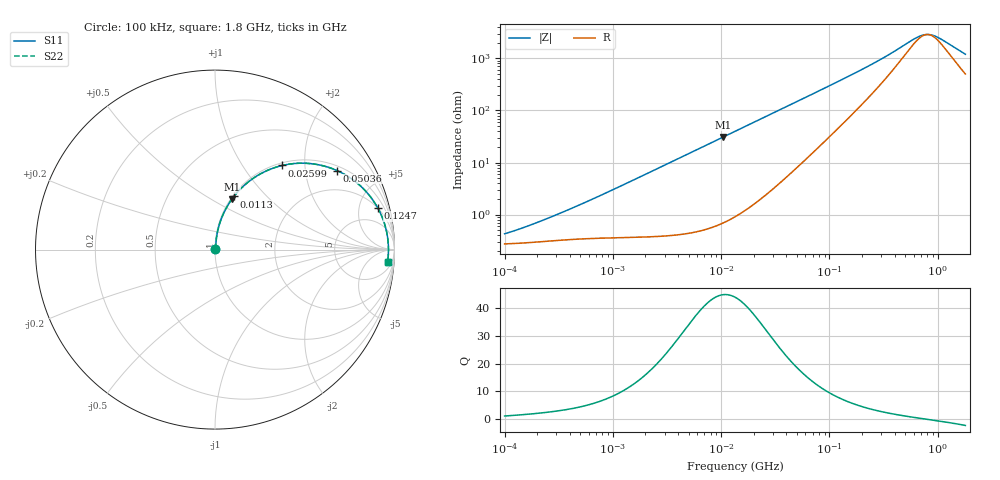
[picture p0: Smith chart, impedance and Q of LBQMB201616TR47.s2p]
! LBQMB201616TR47  S-PARAMETER MODEL  ( General Type )
! Model Generated by TAIYO YUDEN Corporation (http://www.ty-top.com)
! Version 1.0
! TAIYO YUDEN Control No. 191025NI43SB-FBB
! Copyright(c) 2019 TAIYO YUDEN CO.,LTD. All Rights Reserved.
! Product Description (link to TY-COMPAS)
! https://ds.yuden.co.jp/TYCOMPAS/or/detail?pn=LBQMB201616TR47J&u=M
! Products Name : Inductors
! Characteristics :
!  Inductance : 0.47 uH , SRF(min) : 350 MHz , DC Resistance(max) : 0.338 Ohm , Rated Current : 430 mA
!  Case Size : 2.0 x 1.6 / 0.079 x 0.063 [mm/inch] , Thickness : 1.6 / 0.063 [mm/inch]
!  (Conditions: Temperature = 25 degC , DC Bias Current/Voltage = 0A / 0V)
! External Node Assignments :
!  1  o---GGG---o  2
! GND o---------o GND
! Frequency Range : 0.1MHz  -  1800MHz  [ 402 STEP ]
# MHz S RI R 50
! Freq[MHz].  S11 Real  S11 Imag  S21 Real  S21 Imag  S12 Real  S12 Imag  S22 Real  S22 Imag
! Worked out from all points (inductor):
!   401 points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, 100 kHz to 1.8 GHz, reference 50 ohm
!   read as one part in series: L = 489 nH near 308.6 kHz
!   highest Q = 44.7 at 10.5 MHz (marker M1), where L = 470 nH
!   self-resonance near 803.5 MHz
!   S11 on the Smith chart (normalised r, x): 100 kHz: 1.01, +0.01; 11.3 MHz: 1.01, +0.67; 25.99 MHz: 1.05, +1.54; 50.36 MHz: 1.16, +2.98; 124.7 MHz: 1.98, +7.42; 1.8 GHz: 11, -22
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0.1  0.00273 0.00327  0.9973 -0.00327  0.9973 -0.00327  0.00273 0.00327
0.193745  0.00298 0.00616  0.997 -0.00616  0.997 -0.00616  0.00298 0.00616
0.516129  0.00363 0.0155  0.9964 -0.0155  0.9964 -0.0155  0.00363 0.0155
2.66389  0.00989 0.0777  0.9901 -0.0777  0.9901 -0.0777  0.00989 0.0777
5.420303  0.0291 0.1547  0.9709 -0.1547  0.9709 -0.1547  0.0291 0.1547
10.50158  0.0929 0.2794  0.9071 -0.2794  0.9071 -0.2794  0.0929 0.2794
11.30236  0.1056 0.2963  0.8944 -0.2963  0.8944 -0.2963  0.1056 0.2963
13.41641  0.1414 0.3372  0.8586 -0.3372  0.8586 -0.3372  0.1414 0.3372
18.44729  0.2347 0.4113  0.7653 -0.4113  0.7653 -0.4113  0.2347 0.4113
25.99364  0.3749 0.4687  0.6251 -0.4687  0.6251 -0.4687  0.3749 0.4687
35.74074  0.5266 0.4797  0.4734 -0.4797  0.4734 -0.4797  0.5266 0.4797
50.36143  0.6807 0.4399  0.3193 -0.4399  0.3193 -0.4399  0.6807 0.4399
69.24595  0.7918 0.3711  0.2082 -0.3711  0.2082 -0.3711  0.7918 0.3711
90.65972  0.8573 0.3053  0.1427 -0.3053  0.1427 -0.3053  0.8573 0.3053
124.6553  0.9068 0.2323  0.0932 -0.2323  0.0932 -0.2323  0.9068 0.2323
203.4578  0.945 0.1422  0.055 -0.1422  0.055 -0.1422  0.945 0.1422
357.3983  0.9613 0.0706  0.0387 -0.0706  0.0387 -0.0706  0.9613 0.0706
627.8136  0.9661 0.0196  0.0339 -0.0196  0.0339 -0.0196  0.9661 0.0196
709.6131  0.9664 0.00981  0.0336 -0.00981  0.0336 -0.00981  0.9664 0.00981
802.0705  0.9665 0.000143  0.0335 -0.000143  0.0335 -0.000143  0.9665 0.000143
999.899  0.9662 -0.0173  0.0338 0.0173  0.0338 0.0173  0.9662 -0.0173
1800  0.9614 -0.0702  0.0386 0.0702  0.0386 0.0702  0.9614 -0.0702
